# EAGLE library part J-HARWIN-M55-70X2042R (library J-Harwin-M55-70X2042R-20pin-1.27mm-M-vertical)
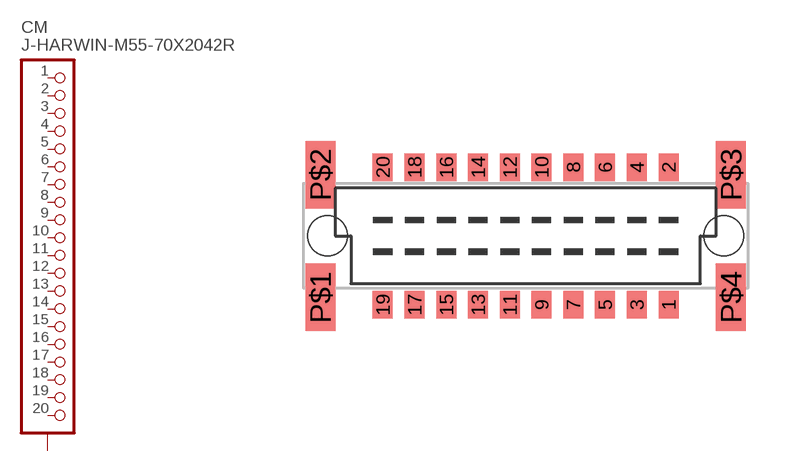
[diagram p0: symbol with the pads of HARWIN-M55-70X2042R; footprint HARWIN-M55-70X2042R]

Designator prefix CM

## J-HARWIN-M55-70X2042R  [HARWIN-M55-70X2042R]
1  1  pas
2  2  pas
3  3  pas
4  4  pas
5  5  pas
6  6  pas
7  7  pas
8  8  pas
9  9  pas
10  10  pas
11  11  pas
12  12  pas
13  13  pas
14  14  pas
15  15  pas
16  16  pas
17  17  pas
18  18  pas
19  19  pas
20  20  pas
P$1  SHIELDS  pas
P$2  SHIELDS  pas
P$3  SHIELDS  pas
P$4  SHIELDS  pas

## Footprint HARWIN-M55-70X2042R (pad centres in mm)
smd 0.8 x 1.1: 1 5.715,-2.75; 2 5.715,2.75; 3 4.445,-2.75; 4 4.445,2.75; 5 3.175,-2.75; 6 3.175,2.75; 7 1.905,-2.75; 8 1.905,2.75; 9 0.635,-2.75; 10 0.635,2.75; 11 -0.635,-2.75; 12 -0.635,2.75; 13 -1.905,-2.75; 14 -1.905,2.75; 15 -3.175,-2.75; 16 -3.175,2.75; 17 -4.445,-2.75; 18 -4.445,2.75; 19 -5.715,-2.75; 20 -5.715,2.75
smd 1.2 x 2.7: P$1 -8.21,-2.45; P$2 -8.21,2.45; P$3 8.21,2.45; P$4 8.21,-2.45
hole 1.6 at -7.925,0
hole 1.6 at 7.925,0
